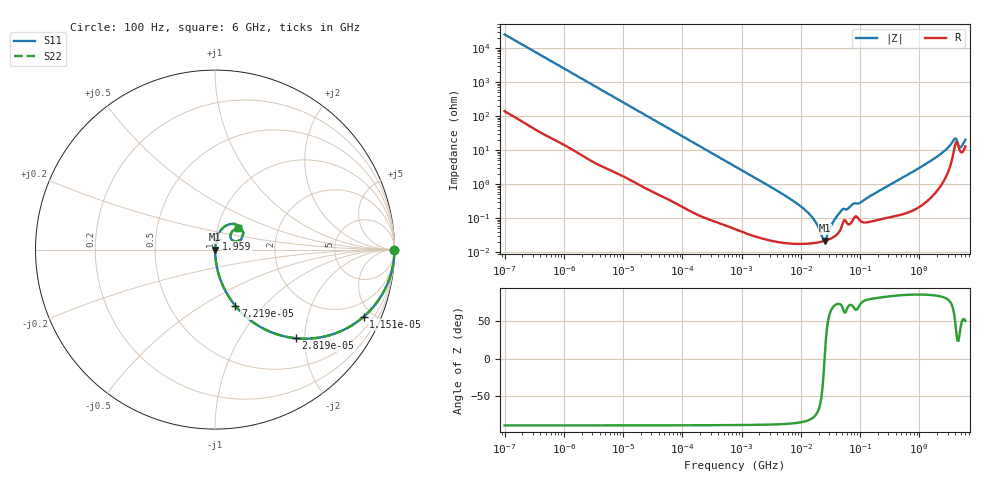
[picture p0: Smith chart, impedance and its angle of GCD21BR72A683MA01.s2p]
!Murata Part Number: GCD21BR72A683MA01
!These Parameters are Measured in Series Mode Connection
!Data Generated on Jan 08, 2026
!  o--ll--o
!Port1  Port2
!  o------o
!Operation Temp=25[degC], DC Bias Voltage=0[V]
!Freq. Start=100[Hz] Stop=6[GHz] 401[Steps]
# Hz S RI R 50
!Freq.(Hz) S11(Real) S11(Imag) S21(Real) S21(Imag) S12(Real) S12(Imag) S22(Real) S22(Imag)
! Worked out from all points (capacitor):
!   401 points, 100 Hz to 6 GHz, reference 50 ohm
!   read as one part in series: C = 63.7 nF near 109 Hz
!   lowest |Z| = 21.7 mohm at 25.46 MHz (marker M1)
!   series resonance near 25.2 MHz, so ESL is about 630 pH
!   S11 on the Smith chart (normalised r, x): 100 Hz: open; 11.51 kHz: 1.03, -4.41; 28.19 kHz: 1.01, -1.81; 72.19 kHz: 1.01, -0.71; 1.959 GHz: 1.01, +0.13; 6 GHz: 1.26, +0.31
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100  1 -0.00401  3.83e-05 0.00401  3.83e-05 0.00401  1 -0.00401
2008  0.9933 -0.0791  0.00674 0.0791  0.00674 0.0791  0.9933 -0.0791
5882  0.9475 -0.22  0.0525 0.22  0.0525 0.22  0.9475 -0.22
11514  0.8276 -0.3743  0.1724 0.3743  0.1724 0.3743  0.8276 -0.3743
28191  0.4498 -0.4939  0.5502 0.4939  0.5502 0.4939  0.4498 -0.4939
40335  0.2872 -0.4487  0.7128 0.4487  0.7128 0.4487  0.2872 -0.4487
72189  0.1136 -0.3133  0.8864 0.3133  0.8864 0.3133  0.1136 -0.3133
202169  0.017 -0.1249  0.983 0.1249  0.983 0.1249  0.017 -0.1249
774597  0.00159 -0.0334  0.9984 0.0334  0.9984 0.0334  0.00159 -0.0334
6644369  0.000193 -0.00367  0.9998 0.00367  0.9998 0.00367  0.000193 -0.00367
1.555665e7  0.000184 -0.00105  0.9998 0.00105  0.9998 0.00105  0.000184 -0.00105
1.86079e7  0.000191 -0.000644  0.9998 0.000644  0.9998 0.000644  0.000191 -0.000644
2.327686e7  0.000207 -0.000167  0.9998 0.000167  0.9998 0.000167  0.000207 -0.000167
2.545746e7  0.000216 2.16e-05  0.9998 -2.16e-05  0.9998 -2.16e-05  0.000216 2.16e-05
3.64232e7  0.000286 0.000811  0.9997 -0.000811  0.9997 -0.000811  0.000286 0.000811
4.983056e7  0.000616 0.00167  0.9994 -0.00167  0.9994 -0.00167  0.000616 0.00167
1.020051e8  0.000833 0.00278  0.9992 -0.00278  0.9992 -0.00278  0.000833 0.00278
3.124326e8  0.00114 0.00925  0.9989 -0.00925  0.9989 -0.00925  0.00114 0.00925
1.95892e9  0.00989 0.0616  0.9901 -0.0616  0.9901 -0.0616  0.00989 0.0616
3.8344e9  0.1089 0.1434  0.8911 -0.1434  0.8911 -0.1434  0.1089 0.1434
5.016141e9  0.0855 0.0698  0.9145 -0.0698  0.9145 -0.0698  0.0855 0.0698
6e9  0.1301 0.1205  0.8699 -0.1205  0.8699 -0.1205  0.1301 0.1205
